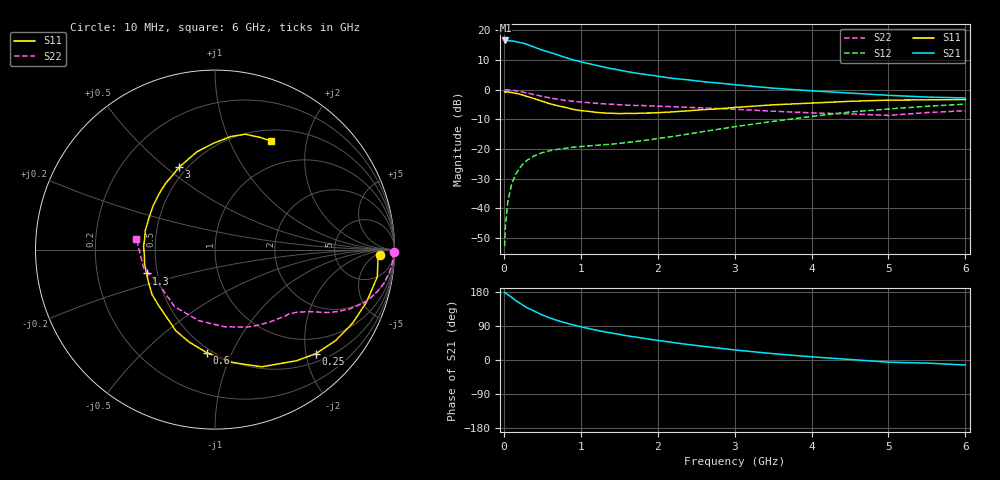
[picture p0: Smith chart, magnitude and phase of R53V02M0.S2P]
! SIEMENS Small Signal Semiconductors
! BFR183
! Si NPN RF Bipolar Junction Transistor in SOT23
! VCE = 3 V  IC = 2 mA
! Common Emitter S-Parameters:  May  1996
# GHz  S  MA  R  50
!  f  S11  S21  S12  S22
! GHz  MAG  ANG  MAG  ANG  MAG  ANG  MAG  ANG
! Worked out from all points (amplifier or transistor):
!   36 points, 10 MHz to 6 GHz, reference 50 ohm
!   highest |S21| = 16.6 dB at 20 MHz (marker M1)
!   |S21| within 3 dB of that: start of sweep to 472.8 MHz
!   unconditionally stable (mu >= 1): 1.389 GHz to 2.826 GHz
!   at 250 MHz: K = 0.23, MSG = 20.3 dB, |S12| = -25.0 dB
!   at 1.4 GHz: K = 1.01, MAG = 12.3 dB, |S12| = -18.4 dB
!   at 6 GHz: K = 0.91, MSG = 1.0 dB, |S12| = -4.9 dB
!   S11 on the Smith chart (normalised r, x): 10 MHz: 20, -8; 250 MHz: 0.66, -2.20; 600 MHz: 0.47, -0.81; 1.3 GHz: 0.43, -0.14; 3 GHz: 0.45, +0.56; 6 GHz: 0.64, +1.44
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0.01  0.9182 -1.9  6.702 178.9  0.0023 92.7  0.9966 -0.8
0.02  0.9097 -3.7  6.746 176.9  0.0048 88.7  0.9905 -1.5
0.05  0.917 -9.5  6.691 172.7  0.0126 84.3  0.9923 -3.9
0.1  0.8938 -18.9  6.62 165.6  0.0251 79.4  0.979 -7.6
0.15  0.8694 -28.1  6.478 157.5  0.0367 73.8  0.9592 -11.3
0.25  0.8072 -45.9  6.068 144.3  0.0564 65.2  0.9069 -17.3
0.3  0.7681 -53.7  5.803 138.2  0.0642 61.6  0.8772 -19.9
0.4  0.7031 -68.2  5.183 128.5  0.0772 55.2  0.8201 -23.8
0.5  0.6361 -81.4  4.632 118.8  0.0867 50.7  0.7691 -26.6
0.6  0.5772 -94.4  4.241 110.9  0.0937 47.2  0.7251 -28.9
0.7  0.5348 -105.6  3.855 104.1  0.0986 45.1  0.689 -30.5
0.8  0.5019 -115.9  3.49 98.0  0.1027 43.3  0.6581 -31.8
0.9  0.4652 -124.9  3.18 92.7  0.1071 42.6  0.6371 -32.9
1.1  0.431 -144.4  2.753 83.2  0.1126 42.1  0.6035 -35.1
1.3  0.4041 -160.8  2.403 74.9  0.1182 43.4  0.5769 -37.1
1.6  0.3984 177.3  2.016 63.8  0.1286 46.5  0.5486 -40.6
2.2  0.4224 144.7  1.548 46.1  0.1632 52.6  0.5148 -49.7
3  0.5005 113.6  1.213 26.6  0.2376 53.7  0.4671 -67.6
3.5  0.5548 100.4  1.059 16.7  0.2917 50.2  0.4331 -83.0
4.5  0.6361 82.1  0.876 1.4  0.4198 38.5  0.3897 -125.3
5.5  0.6732 68.4  0.75 -8.2  0.5244 23.8  0.4103 -165.5
6  0.6812 62.7  0.724 -13.2  0.5699 14.6  0.4417 172.2
